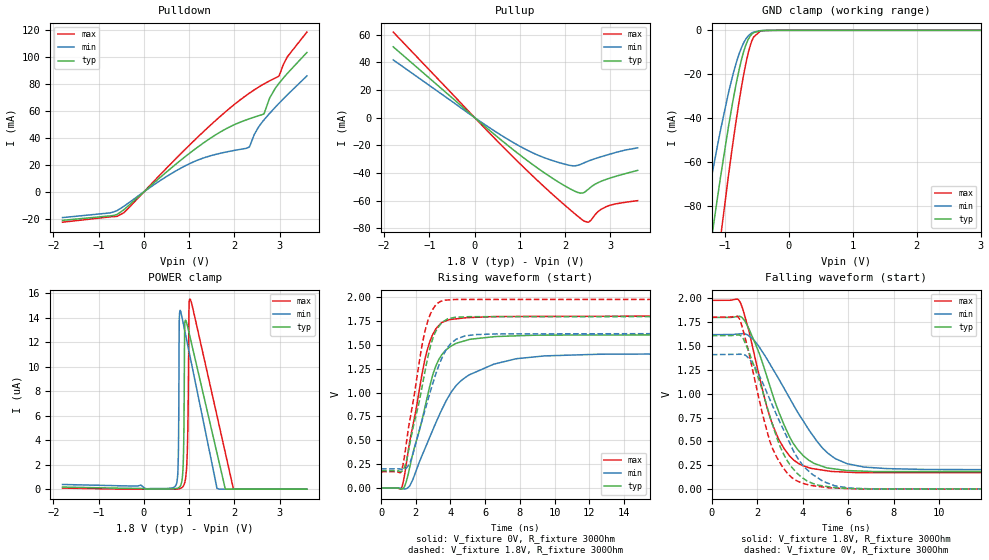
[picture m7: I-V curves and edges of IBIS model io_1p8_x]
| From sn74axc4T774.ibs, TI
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|   io_1p8_x Model
[Model]   io_1p8_x
Model_type   I/O
Polarity   Non-Inverting
Enable   Active-Low
Vinl = 0.63
Vinh = 1.17
Vmeas = 0.9
Vref = 0
Cref = 2pF
Rref = 100000
|   typ   min   max
C_comp   2.803pF   2.059pF   3.293pF
[Model spec]
|subparameter
Vinl   0.63   0.567   0.693
Vinh   1.17   1.053   1.287
| Where Nom  PVT is Nominal Process, 1.8V, 27C
|   Fast PVT is Strong Process,  1.98V, -40C
|   Slow PVT is Weak Process,   1.62V, 130C
[Voltage Range]   1.8   1.62   1.98
|Junction Temperature
[Temperature Range]   27   130   -40
[Pullup Reference]   1.8   1.62   1.98
[Pulldown Reference]   0   0   -0
[Power Clamp Reference]   1.8   1.62   1.98
[GND Clamp Reference]   0   0   0
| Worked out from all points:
|   slope of the pulldown table from 0 to 0.27 V, typ, clamps not added: 33.6 ohm
|   slope of the pullup table from 0 to 0.27 V, typ, clamps not added: 35.7 ohm
|   GND clamp passes 1 mA (typ) near -0.54 V on its own axis
|   falling waveform, V_fixture 1.8V, R_fixture 300Ohm: 20-80 % time 1.52ns typ, 2.19ns min, 1.25ns max; typ from 1.8 V to 0.18 V
|   rising waveform, V_fixture 0V, R_fixture 300Ohm: 20-80 % time 1.4ns typ, 2.4ns min, 1.11ns max; typ from 0 V to 1.61 V
|   rising waveform, V_fixture 1.8V, R_fixture 300Ohm: 20-80 % time 1.13ns typ, 1.42ns min, 993ps max; typ from 0.18 V to 1.8 V
|   falling waveform, V_fixture 0V, R_fixture 300Ohm: 20-80 % time 1.4ns typ, 1.69ns min, 1.18ns max; typ from 1.61 V to 0 V
[Pulldown]
|   Voltage   I(typ)   I(min)   I(max)
-1.8V     -21.17mA   -19.12mA   -22.53mA
-757.8mV  -17.89mA   -15.68mA   -18.62mA
-444.6mV  -13.3mA    -10.8mA    -15.51mA
1.008V    28.56mA    20.82mA    34.65mA
1.748V    45.46mA    28.98mA    57.69mA
2.331V    54.09mA    33.24mA    73.1mA
2.439V    55.32mA    42.55mA    75.54mA
2.65V     57.69mA    53.15mA    79.86mA
2.774V    69.24mA    57.97mA    82.14mA
2.979V    80.14mA    65.37mA    85.6mA
3.173V    87.88mA    72.02mA    100.2mA
3.6V      103.2mA    85.83mA    118.3mA
[GND Clamp]
|   Voltage   I(typ)   I(min)   I(max)
-1.8V     -227.7mA   -173.3mA   -280.5mA
-1.314V   -118.5mA   -85.12mA   -156mA
-1.211V   -96.81mA   -68.22mA   -130.5mA
-1.114V   -76.99mA   -53.06mA   -106.8mA
-1.06V    -66.38mA   -45.06mA   -94mA
-898.2mV  -36.91mA   -23.54mA   -57.37mA
-774mV    -18.07mA   -10.82mA   -32.58mA
-671.4mV  -6.964mA   -4.128mA   -15.65mA
-574.2mV  -1.723mA   -1.197mA   -4.839mA
-444.6mV  -206.1uA   -178.2uA   -421.8uA
-342mV    -62.95uA   -50.11uA   -87.95uA
3.6V      0A         0A         0A
[Pullup]
|   Voltage   I(typ)   I(min)   I(max)
-1.8V     51.17mA    41.74mA    61.84mA
160.2mV   -4.515mA   -3.604mA   -5.474mA
991.8mV   -26.76mA   -20.56mA   -33mA
1.445V    -37.73mA   -27.74mA   -47.19mA
1.975V    -48.96mA   -33.46mA   -62.78mA
2.207V    -53.04mA   -34.78mA   -69.28mA
2.336V    -54.53mA   -33.75mA   -72.75mA
2.401V    -54.26mA   -32.84mA   -74.35mA
2.525V    -51.27mA   -31.15mA   -75.29mA
2.725V    -46.94mA   -28.92mA   -67.84mA
2.984V    -43.68mA   -26.36mA   -63.32mA
3.6V      -38.06mA   -21.81mA   -59.93mA
[POWER Clamp]
|   Voltage   I(typ)   I(min)   I(max)
-1.8V     171.8nA    383.4nA    88.28nA
689.4mV   39.1nA     223nA      568pA
754.2mV   97.12nA    1.895uA    18.8nA
781.2mV   159nA      14.01uA    37.55nA
867.6mV   2.112uA    13.55uA    243nA
900mV     13.42uA    12.97uA    522.5nA
959.4mV   13.35uA    11.9uA     3.252uA
997.2mV   12.76uA    11.22uA    15.28uA
1.013V    12.5uA     10.93uA    15.53uA
1.613V    2.958uA    63.04nA    6.012uA
1.975V    0A         0A         50.55nA
3.6V      0A         0A         0A
[Ramp]
R_load = 300
|   typ   min   max
dV/dt_r   0.965626/1.39522e-09   0.846149/2.40236e-09   1.08236/1.11136e-09
dV/dt_f   0.971927/1.51868e-09   0.851682/2.18327e-09   1.08605/1.24688e-09
[Falling Waveform]
V_fixture = 1.8V
V_fixture_min = 1.62V
V_fixture_max = 1.98V
R_fixture = 300Ohm
C_fixture = 0F
|   Time   V(typ)   V(min)   V(max)
0s        1.8V       1.62V      1.98V
1.255ns   1.81V      1.629V     1.956V
1.932ns   1.514V     1.539V     1.343V
2.546ns   1.086V     1.315V     760.6mV
2.938ns   811.6mV    1.157V     523.6mV
3.405ns   555mV      960.7mV    352mV
4.04ns    346mV      706.6mV    242.7mV
4.889ns   237mV      424.8mV    198.8mV
6.434ns   190.8mV    243.7mV    172.9mV
500ns     180.1mV    200.5mV    169.9mV
[Rising Waveform]
V_fixture = 0V
V_fixture_min = 0V
V_fixture_max = 0V
R_fixture = 300Ohm
C_fixture = 0F
|   Time   V(typ)   V(min)   V(max)
0s        196.5nV    802.5nV    90.45nV
1.209ns   -11.96mV   -5.306mV   11.8mV
1.678ns   236.9mV    30.08mV    511.8mV
2.502ns   824.7mV    400.6mV    1.327V
3.15ns    1.275V     680.3mV    1.665V
4.364ns   1.518V     1.081V     1.774V
6.486ns   1.585V     1.297V     1.796V
12.47ns   1.603V     1.401V     1.799V
31.87ns   1.609V     1.41V      1.804V
500ns     1.609V     1.41V      1.804V
[Rising Waveform]
V_fixture = 1.8V
V_fixture_min = 1.62V
V_fixture_max = 1.98V
R_fixture = 300Ohm
C_fixture = 0F
|   Time   V(typ)   V(min)   V(max)
0s        180.1mV    200.5mV    169.9mV
1.17ns    172.9mV    195.9mV    171.6mV
1.415ns   250mV      203.2mV    411.7mV
1.678ns   478.6mV    268.9mV    731mV
2.361ns   1.058V     705.7mV    1.495V
2.679ns   1.354V     907.7mV    1.742V
3.24ns    1.671V     1.239V     1.932V
4.289ns   1.789V     1.554V     1.976V
27.8ns    1.796V     1.62V      1.976V
500ns     1.8V       1.62V      1.98V
[Falling Waveform]
|Gnd
V_fixture = 0V
V_fixture_min = 0V
V_fixture_max = 0V
R_fixture = 300Ohm
C_fixture = 0F
|   Time   V(typ)   V(min)   V(max)
0s        1.609V     1.41V      1.804V
1.221ns   1.616V     1.414V     1.783V
1.735ns   1.371V     1.34V      1.315V
2.542ns   771.5mV    945.7mV    508.8mV
3.309ns   300.7mV    541.9mV    169.3mV
3.781ns   159.2mV    321.8mV    82.73mV
4.418ns   61.29mV    154.9mV    36.97mV
5.394ns   15.94mV    36.08mV    11.78mV
6.434ns   4.096mV    8.59mV     1.819mV
500ns     208.6nV    855nV      62.14nV
